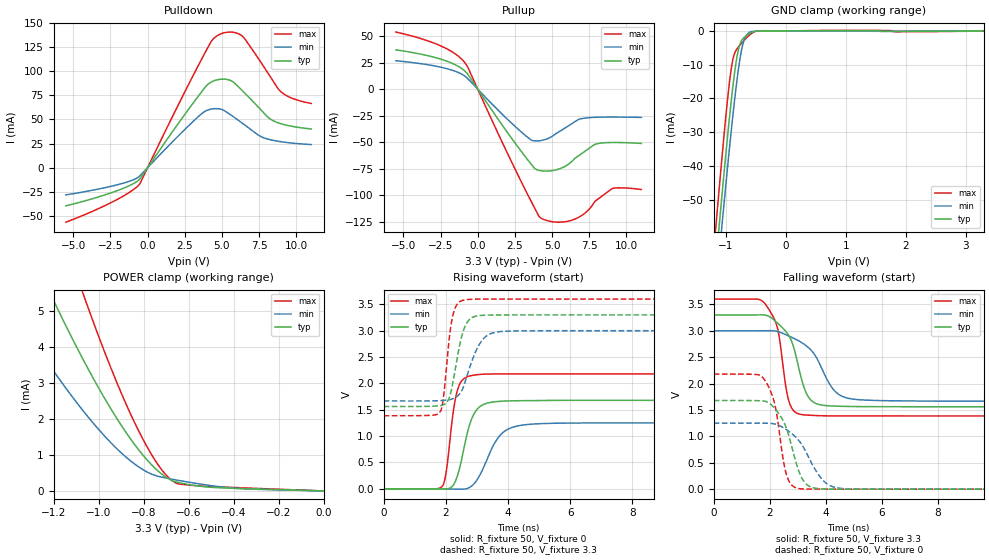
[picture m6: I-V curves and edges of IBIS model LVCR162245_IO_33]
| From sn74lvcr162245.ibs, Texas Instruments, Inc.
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[Model]   LVCR162245_IO_33
Model_type  I/O
Vinl=0.8
Vinh=2.0
Enable   Active-Low
Vref =   0
Rref =   500
Cref =   50p
Vmeas =   1.5
| variable   typ   min   max
C_comp   7.24pF   6.24pF   8.74pF
| C_pullup   5.54pF   4.46pF   7.48pF
| C_pulldown   5.29pF   4.47pF   6.81pF
| C_tri-state   7.24pF   6.24pF   8.74pF
[Temperature Range]   40   100   -40
| Ambient temperature   25   85   -40
[Voltage range]   3.3   3   3.6
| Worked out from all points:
|   slope of the pulldown table from 0 to 0.495 V, typ, clamps not added: 44.3 ohm
|   slope of the pullup table from 0 to 0.495 V, typ, clamps not added: 47.6 ohm
|   GND clamp passes 1 mA (typ) near -0.62 V on its own axis
|   POWER clamp passes 1 mA (typ) near -0.80 V on its own axis
|   rising waveform, R_fixture 50, V_fixture 0: 20-80 % time 426ps typ, 640ps min, 282ps max; typ from 0 V to 1.68 V
|   falling waveform, R_fixture 50, V_fixture 3.3: 20-80 % time 611ps typ, 948ps min, 397ps max; typ from 3.3 V to 1.56 V
|   rising waveform, R_fixture 50, V_fixture 3.3: 20-80 % time 347ps typ, 504ps min, 239ps max; typ from 1.56 V to 3.3 V
|   falling waveform, R_fixture 50, V_fixture 0: 20-80 % time 613ps typ, 875ps min, 415ps max; typ from 1.68 V to 0 V
[GND Clamp]
| LVCR162245_IO_33
|   Voltage   I(typ)   I(min)   I(max)
-5.5V     -1A        -986.7mA   -1.023A
-1.185V   -72.48mA   -81mA      -62.07mA
-1.155V   -66.51mA   -75.16mA   -55.89mA
-1.105V   -56.67mA   -65.52mA   -45.74mA
-1.085V   -52.78mA   -61.7mA    -41.75mA
-1.06V    -47.97mA   -56.96mA   -36.84mA
-950mV    -27.71mA   -36.77mA   -17mA
-885mV    -17mA      -25.62mA   -8.785mA
-805mV    -6.9mA     -13.45mA   -5.118mA
-740mV    -3.004mA   -5.959mA   -3.721mA
-615mV    -934.8uA   -567.9uA   -1.427mA
3.3V      73.49pA    45.03uA    -66.26uA
[POWER Clamp]
| LVCR162245_IO_33
|   Voltage   I(typ)   I(min)   I(max)
-5.5V     84.14mA    60.03mA    122mA
-1.42V    8.324mA    5.427mA    12.4mA
-1.215V   5.482mA    3.461mA    8.205mA
-1.085V   3.842mA    2.354mA    5.767mA
-1.06V    3.546mA    2.157mA    5.323mA
-920mV    2.024mA    1.18mA     3.027mA
-820mV    1.128mA    660.2uA    1.645mA
-735mV    550.2uA    404.3uA    723.1uA
-675mV    294.3uA    327.3uA    294.7uA
-640mV    227.4uA    287.2uA    189.6uA
-390mV    71.22uA    71.66uA    93.3uA
-95.1fV   73.49pA    196pA      354.1pA
[Pulldown]
| LVCR162245_IO_33
|   Voltage   I(typ)   I(min)   I(max)
-5.5V     -39.6mA    -28.23mA   -56.53mA
-2.325V   -25.38mA   -18.82mA   -35.2mA
-575mV    -12.59mA   -9.301mA   -17.77mA
3.585V    77.77mA    55.34mA    111.2mA
4.295V    88.99mA    60.81mA    131.4mA
4.825V    91.58mA    61.01mA    138.1mA
5.62V     90.17mA    54.41mA    140.6mA
6.325V    80.55mA    46.67mA    137mA
7.615V    60.04mA    32.28mA    109.3mA
8.205V    50.92mA    29.17mA    95.43mA
8.905V    45.91mA    27.08mA    79.6mA
11V       40.14mA    23.97mA    66.64mA
[Pullup]
| LVCR162245_IO_33
|   Voltage   I(typ)   I(min)   I(max)
-5.5V     37.13mA    26.85mA    53.89mA
-2.51V    28.45mA    20.84mA    41.02mA
-1.52V    23.1mA     16.95mA    33.4mA
-860mV    17.04mA    12.27mA    24.89mA
3.13V     -62.49mA   -42.82mA   -93.1mA
3.82V     -74.71mA   -48.76mA   -112.1mA
4.25V     -77.01mA   -48.48mA   -121.7mA
5.64V     -74.4mA    -38.69mA   -125.5mA
6.95V     -61.21mA   -27.91mA   -119.6mA
7.905V    -52.01mA   -26.56mA   -105.6mA
9.045V    -50.33mA   -26.31mA   -93.85mA
11V       -51.22mA   -26.66mA   -94.71mA
[Ramp]
| LVCR162245_IO_33
| variable   typ   min   max
dV/dt_r   1.01/4.28E-10   0.75/6.47E-10   1.31/2.83E-10
dV/dt_f   1.04/6.15E-10   0.80/9.55E-10   1.33/4.01E-10
R_load = 50
[Rising Waveform]
| LVCR162245_IO_33
R_fixture =   50
C_fixture =   0
L_fixture =   0
V_fixture =   0
V_fixture_min = 0
V_fixture_max = 0
|   Time   V(typ)   V(min)   V(max)
0s        489.6pV    1.24nV     4.34nV
1.89ns    -2.767mV   -1.631mV   54.23mV
2.01ns    -111.2uV   -2.134mV   321.7mV
2.235ns   68.88mV    -3.514mV   1.449V
2.37ns    245.1mV    -5.079mV   1.866V
2.72ns    1.127V     14.83mV    2.133V
2.91ns    1.428V     99.96mV    2.158V
3.755ns   1.661V     1.023V     2.18V
4.675ns   1.673V     1.224V     2.18V
24.99ns   1.679V     1.251V     2.18V
[Falling Waveform]
| LVCR162245_IO_33
R_fixture =   50
C_fixture =   0
L_fixture =   0
V_fixture =   3.3
V_fixture_min = 3
V_fixture_max = 3.6
|   Time   V(typ)   V(min)   V(max)
0s        3.3V       3V         3.6V
1.86ns    3.294V     3.002V     3.491V
2.285ns   3.141V     2.986V     3.022V
2.565ns   2.991V     2.928V     1.958V
2.69ns    2.896V     2.898V     1.65V
3.115ns   2.117V     2.783V     1.415V
3.6ns     1.634V     2.546V     1.396V
4.31ns    1.574V     1.863V     1.388V
5.085ns   1.565V     1.699V     1.387V
24.99ns   1.562V     1.667V     1.387V
[Rising Waveform]
| LVCR162245_IO_33
R_fixture =   50
C_fixture =   0
L_fixture =   0
V_fixture =   3.3
V_fixture_min = 3
V_fixture_max = 3.6
|   Time   V(typ)   V(min)   V(max)
0s        1.562V     1.667V     1.387V
1.81ns    1.578V     1.674V     1.457V
1.92ns    1.593V     1.678V     1.725V
2.11ns    1.724V     1.691V     2.855V
2.22ns    1.999V     1.709V     3.276V
2.46ns    2.77V      1.817V     3.555V
2.625ns   3.094V     2.038V     3.586V
3.145ns   3.29V      2.802V     3.599V
3.815ns   3.299V     2.986V     3.6V
24.99ns   3.3V       3V         3.6V
[Falling Waveform]
| LVCR162245_IO_33
R_fixture =   50
C_fixture =   0
L_fixture =   0
V_fixture =   0
V_fixture_min = 0
V_fixture_max = 0
|   Time   V(typ)   V(min)   V(max)
0s        1.679V     1.251V     2.18V
1.805ns   1.668V     1.249V     2.077V
2.18ns    1.526V     1.234V     1.599V
2.47ns    1.3V       1.168V     582mV
2.6ns     1.141V     1.124V     261.6mV
3.04ns    333.2mV    916.9mV    11.21mV
3.335ns   80.05mV    655.7mV    1.519mV
3.885ns   4.386mV    175.1mV    342.6uV
4.615ns   604.7uV    10.62mV    75.92uV
24.99ns   1.672uV    1.308uV    948.1nV
